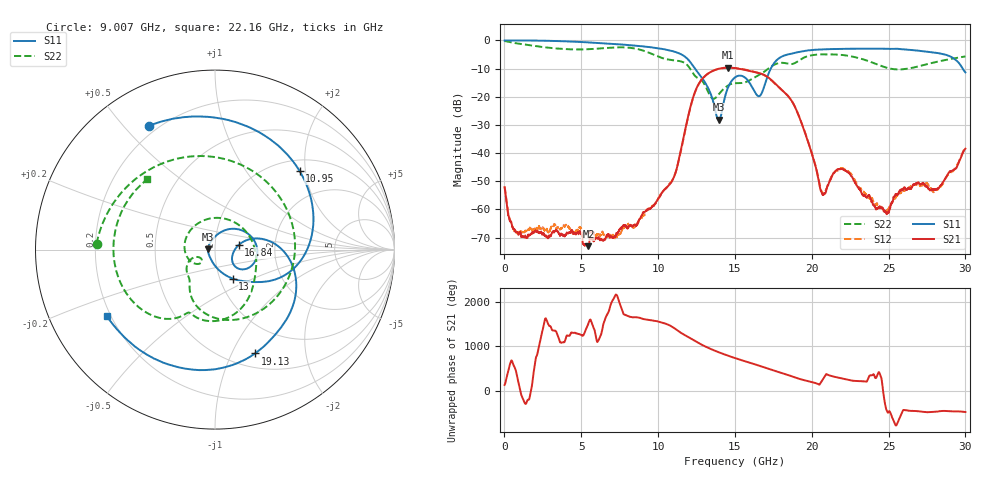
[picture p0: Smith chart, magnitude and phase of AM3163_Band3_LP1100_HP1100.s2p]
!Agilent Technologies,E8364B,MY43040894,A.07.50.67
!Agilent E8364B: A.07.50.67
!Date: Thursday, August 20, 2020 11:07:22
!Correction: S11(Full 2 Port(1,2))
!S21(Full 2 Port(1,2))
!S12(Full 2 Port(1,2))
!S22(Full 2 Port(1,2))
!S2P File: Measurements: S11, S21, S12, S22:
# Hz S  dB  R 50
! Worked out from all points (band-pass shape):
!   3201 points, 10 MHz to 30 GHz, reference 50 ohm
!   highest |S21| = -9.66 dB at 14.56 GHz (marker M1); lowest = -73.0 dB at 5.464 GHz (marker M2)
!   |S21| within 3 dB of the highest: 13.05 GHz to 17.03 GHz (3.98 GHz wide, 26.5 % of centre)
!   lowest |S11| = -28.2 dB at 13.95 GHz (marker M3), VSWR 1.08, Z = 46.2 + j0.185 ohm
!   |S11| at or under -10 dB: 12.4 GHz to 17.34 GHz (4.939 GHz wide, 33.2 % of centre); 29.82 GHz to end of sweep
!   |S22| runs from -20.7 to -0.2 dB; largest |S21 - S12| = 0.0078
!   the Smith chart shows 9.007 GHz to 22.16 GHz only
!   S11 on the Smith chart (normalised r, x): 9.007 GHz: 0.17, +0.59; 10.95 GHz: 1.24, +1.86; 13 GHz: 1.15, -0.39; 16.84 GHz: 1.30, +0.07; 19.13 GHz: 0.66, -1.23; 22.16 GHz: 0.19, -0.28
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1e7  -0.06 -1.8  -52.19 128.0  -51.77 176.4  -0.23 -6.0
1.162741e9  -0.05 -31.3  -69.42 -151.3  -68.12 -48.0  -1.40 -83.6
2.531034e9  -0.14 -67.8  -68.38 -5.6  -66.93 172.9  -2.42 -164.7
5.014581e9  -0.60 -132.0  -68.80 172.3  -67.22 133.4  -3.22 64.8
5.464431e9  -0.72 -143.6  -73.01 76.3  -68.31 -85.9  -3.14 40.3
6.504709e9  -1.06 -170.5  -70.61 126.1  -69.23 15.4  -2.75 -18.6
7.544988e9  -1.45 161.6  -66.87 124.9  -68.50 -34.5  -2.47 -81.4
9.007e9  -2.14 117.9  -61.20 177.2  -62.21 -176.6  -3.60 177.2
1.000979e10  -2.82 82.6  -56.21 116.8  -56.15 118.0  -5.76 90.1
1.094698e10  -3.83 42.9  -49.47 -7.1  -49.38 -8.3  -7.04 -3.9
1.299942e10  -14.46 -58.6  -12.94 -72.8  -12.95 -71.8  -15.40 -153.2
1.394598e10  -28.16 177.1  -10.08 144.9  -10.12 145.1  -19.16 -136.9
1.455515e10  -16.70 52.2  -9.66 66.8  -9.77 67.6  -16.01 -162.3
1.5005e10  -13.15 16.0  -9.82 13.4  -9.85 14.8  -15.20 157.4
1.684189e10  -17.41 11.0  -12.10 171.5  -12.19 171.3  -11.38 -34.5
1.912862e10  -4.15 -68.9  -26.39 -89.0  -26.30 -87.7  -7.30 -118.6
2.000958e10  -3.42 -95.4  -40.26 -167.0  -40.03 -165.6  -5.28 -149.3
2.074059e10  -3.19 -114.8  -54.76 -97.1  -54.45 60.6  -4.95 -175.3
2.215574e10  -3.01 -148.2  -46.05 -101.4  -45.64 -105.2  -5.30 133.9
2.500479e10  -3.02 145.6  -61.18 -117.6  -59.91 24.7  -9.92 -9.3
2.733839e10  -3.93 80.8  -51.11 -121.9  -51.16 -124.3  -8.69 -143.1
3e10  -11.36 -22.6  -38.45 -122.7  -37.92 -119.2  -5.74 118.6
